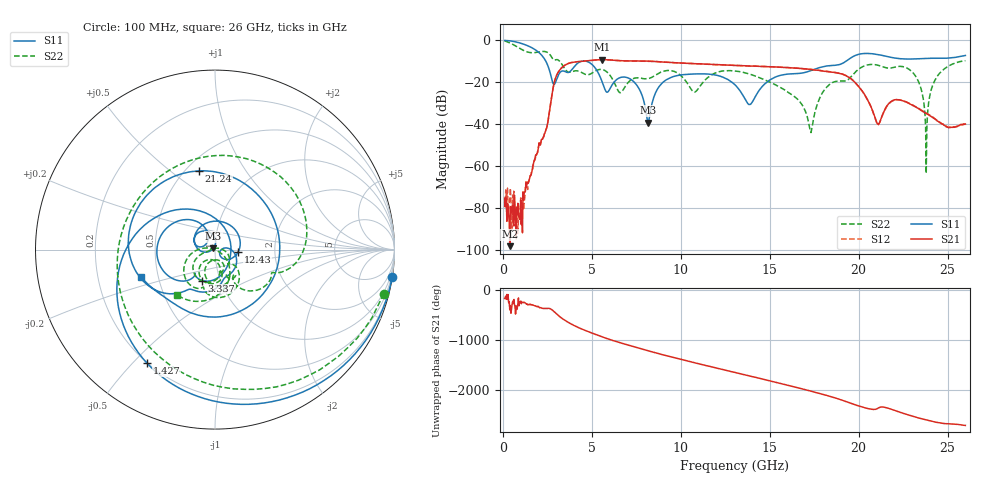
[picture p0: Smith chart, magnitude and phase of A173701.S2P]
!  2-Port S-parameters saved by WinCal
! VAR MeasName=S-Parameters (CALIBRATED_DATA) read from VNA (N5245A)
! VAR MeasDate=2017-6-7 10:28:25
! VAR NAME=A173701
! VAR FILENAME=A173701.S2P
! VAR DATE=2017-6-7 10:28:25
! VAR PHYS_PORTS=1,2
# Hz S DB R 50
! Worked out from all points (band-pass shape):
!   801 points, 100 MHz to 26 GHz, reference 50 ohm
!   highest |S21| = -9.12 dB at 5.571 GHz (marker M1); lowest = -98.0 dB at 391.4 MHz (marker M2)
!   |S21| within 3 dB of the highest: 3.435 GHz to 13.7 GHz (10.27 GHz wide, 120 % of centre)
!   lowest |S11| = -39.1 dB at 8.161 GHz (marker M3), VSWR 1.02, Z = 49.2 + j0.71 ohm
!   |S11| at or under -10 dB: 2.422 GHz to 4.394 GHz (1.972 GHz wide, 57.9 % of centre); 4.723 GHz to 19.28 GHz (14.55 GHz wide, 121 % of centre)
!   |S22| runs from -63.4 to -0.2 dB; largest |S21 - S12| = 0.0038
!   S11 on the Smith chart (normalised r, x): 100 MHz: 0, -13; 1.427 GHz: 0.20, -0.55; 3.337 GHz: 0.82, -0.29; 12.43 GHz: 1.30, -0.03; 21.24 GHz: 0.58, +0.64; 26 GHz: 0.40, -0.15
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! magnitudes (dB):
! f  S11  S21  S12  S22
! 100 MHz  0.0  -75.1  -76.9  -0.2
! 391.4 MHz  -0.2  -98.0  -75.4  -1.2
! 1.071 GHz  -1.5  -81.0  -77.5  -4.4
! 1.427 GHz  -2.6  -68.0  -67.2  -5.6
! 3.337 GHz  -14.6  -12.8  -12.8  -11.5
! 4.438 GHz  -9.9  -10.0  -10.0  -15.3
! 5.571 GHz  -19.5  -9.1  -9.2  -13.8
! 7.255 GHz  -18.9  -9.8  -9.8  -18.5
! 8.161 GHz  -39.1  -9.9  -9.9  -18.2
! 8.744 GHz  -22.5  -10.1  -10.1  -15.7
! 10.78 GHz  -16.0  -11.1  -11.1  -24.6
! 12.43 GHz  -17.7  -11.7  -11.7  -14.5
! 13.05 GHz  -21.2  -11.9  -11.9  -14.6
! 13.89 GHz  -30.5  -12.2  -12.2  -16.1
! 17.39 GHz  -14.2  -14.0  -13.8  -41.0
! 18.33 GHz  -12.0  -14.9  -14.9  -21.3
! 21.24 GHz  -7.0  -37.6  -37.8  -12.2
! 21.69 GHz  -7.8  -30.0  -30.3  -13.2
! 23.15 GHz  -8.8  -31.4  -31.3  -16.4
! 23.8 GHz  -8.6  -34.8  -34.6  -63.4
! 24.41 GHz  -8.5  -38.3  -38.1  -17.2
! 26 GHz  -7.2  -39.8  -39.9  -9.7
